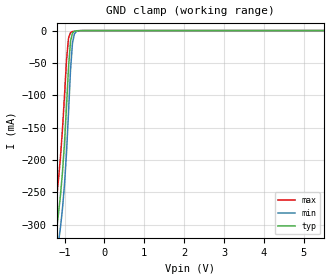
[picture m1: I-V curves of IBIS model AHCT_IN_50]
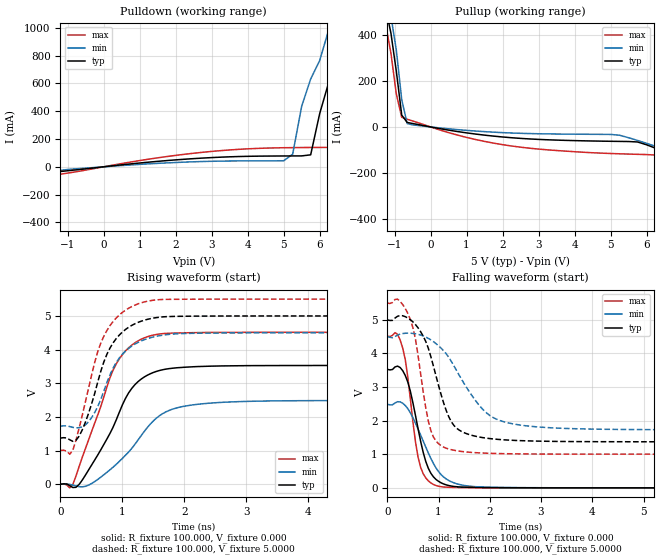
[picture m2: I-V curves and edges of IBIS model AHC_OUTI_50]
| Philips Semiconductors Inc.
| Logic Products Group
| IBIS model of 74AHCT04
| HEX INVERTER; TTL
|[Packages]:
|[Package1]: SO 14-pin (D) Package ;
|[Package2]: TSSOP 14-pin (PW) Package ;
[IBIS Ver]   3.2
[File Name]   ahct04.ibs
[File Rev]   1.4
[Date]   08-Apr-2003
[Source]   File created from simulations by LPG
   Philips Semiconductors Nijmegen
[Notes]   V1.4   Ibis model.
| Remark:
| The Power Clamp curves for the input models have been omitted since there
| is no power clamp diode.
| Revision History
| Version Date   Author/ Description
|   Editor
| 1.3   December   2000 RM   Reviewed version for IBIS 3.2
| 1.4   April   2003 RM   Updated version
[Disclaimer]
   (C) Copyright 2003 Philips Semiconductors
   All rights reserved
   Philips Semiconductors warrants and represents that the IBIS model
   identified herein is owned by Philips Semiconductors (PHILIPS). The
   model provided is not warranted as fully representing all of the
   operating characteristics and specifications of the semiconductor
   products to which the model relates.  Moreover, unless there is a
   signed, written agreement to the contrary, this IBIS model is
   furnished on an "as is" basis without support or warranty of any
   kind, either expressed or implied, regarding the use thereof, and
   PHILIPS specifically disclaims all implied warranties of
   merchantability and fitness of the model for any purpose.
   PHILIPS does not assume any liability arising out of the application
   or use of this IBIS model including infringement of patents and
   copyrights, nor does PHILIPS convey any license under its patents and
   copyrights or the rights of others.
   PHILIPS provides IBIS models as a service to our customers. You and
   your company shall not distribute, convey, sell, or give these models
   to anyone else without receiving prior written permission from
   PHILIPS.
   PHILIPS reserves the right to make changes without notice to these
   IBIS models to improve reliability, function, or design.
   Please be aware that your receipt and subsequent use of the IBIS
   information provided shall serve as acceptance of the terms and
   conditions of this agreement.  If you do not accept these terms,
   you should return or destroy the IBIS models and any other
   accompanying information immediately.
| to specify a consistent format that can be parsed by software, allowing
| simulation vendors to derive models compatible with their own products.
| One goal of this template is to represent the current state of IBIS data,
| while allowing a growth path to more complex models / methods (when deemed
| appropriate).  This would be accomplished by a revision of the base
| template, and possibly the addition of new keywords or categories.
| Another goal of this template is to ensure that it is simple enough for
| semiconductor vendors and customers to use and modify, while ensuring that
| it is rigid enough for simulation vendors to write reliable parsers.
| Finally, this template is meant to contain a complete description of the I/O
| elements on an entire component.  Consequently, several models will need to
| be defined in each file, as well as a table that equates the appropriate
| buffer to the correct pin and signal name.
| Version 3.2 of this electronic template was finalized by an industry-wide
| group of experts representing various companies and interests.  Regular
| "EIA IBIS Open Forum" meetings were held to accomplish this task.
| Commitment to Backward Compatibility.  Version 1.0 is the first valid IBIS
| ASCII file format.  It represents the minimum amount of I/O buffer
| information required to create an accurate IBIS model of common CMOS and
| bipolar I/O structures.  Future revisions of the ASCII file will add items
| considered to be "enhancements" to Version 1.0 to allow accurate modeling
| of new, or other I/O buffer structures.  Consequently, all future revisions
| will be considered supersets of Version 1.0, allowing backward
| compatibility.  In addition, as modeling platforms develop support for
| revisions of the IBIS ASCII template, all previous revisions of the template
| must also be supported.
| Version 1.1 update.  The file "ver1_1.ibs" is conceptually the same as the
| 1.0 version of the IBIS ASCII format (ver1_0.ibs).  However, various
| comments have been added for further clarification.
| Version 2.0 update.  The file "ver2_0.ibs" maintains backward compatibility
| with Versions 1.0 and 1.1.  All new keywords and elements added in Version
| 2.0 are optional.  A complete list of changes to the specification is in the
| IBIS Version 2.0 Release Notes document ("ver2_0.rn").
| Version 2.1 update.  The file "ver2_1.ibs" contains clarification text
| changes, corrections, and two additional waveform parameters beyond
| Version 2.0.
| Version 3.0 update.  The file "ver3_0.ibs" adds a number of new keywords
| and functionality.  A complete list of functions can be found on eda.org
| under /pub/ibis/birds/birddir.txt showing the approved Buffer Issue
| Resolution Documents (BIRDs) that have been approved for Version 3.0.
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[Component]   74AHCT04_1
[Manufacturer]   Philips Semiconductors Inc.
[Package]
|   typ   min   max
R_pkg   4.54E-02   4.18E-02   5.01E-02
L_pkg   2.31E-09   1.63E-09   3.26E-09
C_pkg   0.565E-12  0.437E-12  0.736E-12
[Pin] signal_name   model_name   R_pin   L_pin   C_pin
   1   1A   AHCT_IN_50 4.18E-02 3.26E-09 0.675E-12
   2   1Y#   AHC_OUTI_50 5.01E-02 2.30E-09 0.574E-12
   3   2A   AHCT_IN_50 4.52E-02 1.71E-09 0.467E-12
   4   2Y#   AHC_OUTI_50 4.38E-02 1.63E-09 0.437E-12
   5   3A   AHCT_IN_50 4.52E-02 1.71E-09 0.465E-12
   6   3Y#   AHC_OUTI_50 5.01E-02 2.30E-09 0.573E-12
   7   GND   GND 4.18E-02 3.26E-09 0.736E-12
   8   4Y#   AHC_OUTI_50 4.18E-02 3.26E-09 0.736E-12
   9   4A   AHCT_IN_50 5.01E-02 2.30E-09 0.573E-12
   10   5Y#   AHC_OUTI_50 4.52E-02 1.71E-09 0.465E-12
   11   5A   AHCT_IN_50 4.38E-02 1.63E-09 0.437E-12
   12   6Y#   AHC_OUTI_50 4.52E-02 1.71E-09 0.467E-12
   13   6A   AHCT_IN_50 5.01E-02 2.30E-09 0.574E-12
   14   VCC   POWER 4.18E-02 3.26E-09 0.736E-12
|   Info for  TSSOP 14-pin (PW) Package
[Component]   74AHCT04_2
[Manufacturer]   Philips Semiconductors Inc.
[Package]
|   typ   min   max
R_pkg   3.44E-02   2.80E-02   4.33E-02
L_pkg   1.83E-09   1.36E-09   2.32E-09
C_pkg   0.380E-12  0.302E-12  0.442E-12
[Pin] signal_name   model_name   R_pin   L_pin   C_pin
   1   1A   AHCT_IN_50 3.46E-02 2.32E-09 0.423E-12
   2   1Y#   AHC_OUTI_50 4.33E-02 2.04E-09 0.441E-12
   3   2A   AHCT_IN_50 2.80E-02 1.36E-09 0.307E-12
   4   2Y#   AHC_OUTI_50 2.88E-02 1.38E-09 0.302E-12
   5   3A   AHCT_IN_50 2.80E-02 1.36E-09 0.308E-12
   6   3Y#   AHC_OUTI_50 4.33E-02 2.04E-09 0.441E-12
   7   GND   GND 3.46E-02 2.32E-09 0.433E-12
   8   4Y#   AHC_OUTI_50 3.46E-02 2.32E-09 0.433E-12
   9   4A   AHCT_IN_50 4.33E-02 2.04E-09 0.441E-12
   10   5Y#   AHC_OUTI_50 2.80E-02 1.36E-09 0.308E-12
   11   5A   AHCT_IN_50 2.88E-02 1.38E-09 0.302E-12
   12   6Y#   AHC_OUTI_50 2.80E-02 1.36E-09 0.308E-12
   13   6A   AHCT_IN_50 4.33E-02 2.04E-09 0.442E-12
   14   VCC   POWER 3.46E-02 2.31E-09 0.433E-12
| Models and submodels in the file (2): AHCT_IN_50 (Input), AHC_OUTI_50 (Output)
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|   Model AHCT_IN_50
[Model]   AHCT_IN_50
Model_type   Input
Vinl =   0.8000V
Vinh =   2.0000V
C_comp   5.6pF   4.9pF   6.8pF
[Model Spec]
| Note: The input and output voltage ratings may be exceeded if the input and
|   output current ratings are observed (please refer to the data sheet)
|   Subparameter   typ   min   max
| Thresholds
Vinh   2.0   NA   NA
Vinl   0.8   NA   NA
| Overshoot
S_overshoot_high   7.0   7.0   7.0   | Static overshoot
S_overshoot_low   -0.5   -0.5   -0.5
D_overshoot_high   11.0   11.0   11.0   | Dynamic overshoot
D_overshoot_low   -0.95   -0.9   -1.0
D_overshoot_time   3n   3n   3n
|Ambient temperature:   25.0000   85.0000   -40.0000
[Temperature Range]   55.0000   110.0000   -5.0000
[Voltage Range]   5.0000V   4.5000V   5.5000V
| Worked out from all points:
|   GND clamp passes 1 mA (typ) near -0.75 V on its own axis
|Process Range   nominal   slow   fast
[GND Clamp]
| voltage   I(typ)   I(min)   I(max)
-5.5V     -4.525A    -4.549A    -4.495A
-1.3V     -373.3mA   -409.5mA   -330.1mA
-1.2V     -307.7mA   -348mA     -259.7mA
-1.1V     -253.8mA   -303.6mA   -194.6mA
-1.05V    -218.4mA   -274.7mA   -152mA
-950mV    -118.1mA   -189.3mA   -46.31mA
-900mV    -57.87mA   -127.6mA   -11.93mA
-850mV    -16.96mA   -61.59mA   -3.088mA
-800mV    -3.834mA   -19.15mA   -1.465mA
-750mV    -1.005mA   -4.867mA   -923uA
-600mV    -83.72uA   -113.1uA   -151.7uA
5.5V      58.3pA     1.82nA     103.7fA
|   Model AHC_OUTI_50
[Model]   AHC_OUTI_50
Model_type   Output
Polarity   Inverting
Vmeas =  2.5000V
Cref  = 50.0000pF
Rref  =  1.0000k
Vref  =  0.000V
C_comp   9.0pF   6.7pF   13.1pF
[Model Spec]
| Note: The input and output voltage ratings may be exceeded if the input and
|   output current ratings are observed (please refer to the data sheet)
|   Subparameter   typ   min   max
| Timing Thresholds
Vmeas   2.5   2.25   2.75
|Ambient temperature:   25.0000   85.0000   -40.0000
[Temperature Range]   55.0000   110.0000   -5.0000
[Voltage Range]   5.0000V   4.5000V   5.5000V
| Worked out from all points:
|   slope of the pulldown table from 0 to 0.75 V, typ, clamps not added: 35.9 ohm
|   slope of the pullup table from 0 to 0.75 V, typ, clamps not added: 37.2 ohm
|   rising waveform, R_fixture 100.000, V_fixture 0.000: 20-80 % time 593ps typ, 724ps min, 540ps max; typ from 0 V to 3.53 V
|   rising waveform, R_fixture 100.000, V_fixture 5.0000: 20-80 % time 427ps typ, 449ps min, 428ps max; typ from 1.37 V to 5 V
|   falling waveform, R_fixture 100.000, V_fixture 0.000: 20-80 % time 313ps typ, 464ps min, 232ps max; typ from 3.53 V to 0 V
|   falling waveform, R_fixture 100.000, V_fixture 5.0000: 20-80 % time 435ps typ, 728ps min, 292ps max; typ from 5 V to 1.37 V
|Process Range   nominal   slow   fast
[Pulldown]
| voltage   I(typ)   I(min)   I(max)
-5.5V     -304.7mA   -244.4mA   -420.6mA
-1.6V     -52.82mA   -44.3mA    -71.19mA
2.25V     54.55mA    33.73mA    90.24mA
5V        77.97mA    43.25mA    137.3mA
5.25V     78.26mA    90.83mA    138mA
5.5V      78.46mA    436mA      138.7mA
5.75V     86.23mA    632.3mA    139.2mA
6V        382.8mA    765.2mA    139.3mA
6.25V     606.6mA    985.4mA    139.5mA
6.75V     978.5mA    1.479A     593.9mA
7.25V     1.477A     1.981A     988mA
11V       5.298A     5.791A     4.82A
[Pullup]
| voltage   I(typ)   I(min)   I(max)
-6.5V     5.717A     5.741A     5.691A
-1.25V    521.9mA    583.1mA    449.8mA
-1.1V     409.1mA    483.8mA    321.7mA
-950mV    242.7mA    334.7mA    143.7mA
-800mV    51.78mA    119.1mA    42mA
-650mV    19.63mA    14.69mA    33.56mA
2V        -43.78mA   -24.8mA    -77.21mA
5V        -62.56mA   -32.65mA   -115.8mA
5.75V     -65.59mA   -58.92mA   -119.4mA
6.5V      -108.9mA   -97.5mA    -134mA
9.75V     -328.6mA   -269.4mA   -442.8mA
11V       -414.1mA   -336.1mA   -565.4mA
[Ramp]
| variable   typ   min   max
dV/dt_r   2.117V/593.251ps   1.493V/724.062ps   2.708V/539.812ps
dV/dt_f   2.177V/434.826ps   1.664V/728.595ps   2.698V/291.947ps
R_load = 100.000
[Rising Waveform]
R_fixture   = 100.000
V_fixture   = 0.000
V_fixture_min = 0.000
V_fixture_max = 0.000
| time   V(typ)   V(min)   V(max)
0s        402.7pV    18.45nV    554fV
200ps     -98.16mV   -25.59mV   -9.537mV
300ps     -9.255mV   -71.27mV   519mV
450ps     411.2mV    -30.31mV   1.297V
900ps     1.909V     590.1mV    3.574V
1.15ns    2.845V     1.063V     4.132V
1.45ns    3.282V     1.786V     4.409V
1.85ns    3.455V     2.254V     4.492V
2.65ns    3.516V     2.437V     4.511V
9.75ns    3.528V     2.488V     4.514V
[Rising Waveform]
R_fixture   = 100.000
V_fixture   = 5.0000
V_fixture_min = 4.5000
V_fixture_max = 5.5000
| time   V(typ)   V(min)   V(max)
0s        1.371V     1.726V     1.003V
150ps     1.321V     1.713V     892.4mV
300ps     1.424V     1.679V     1.657V
450ps     2.088V     1.85V      2.823V
600ps     3.022V     2.301V     3.927V
750ps     3.862V     3.023V     4.57V
1ns       4.522V     3.863V     5.106V
1.35ns    4.872V     4.292V     5.415V
2.25ns    4.995V     4.488V     5.498V
9.75ns    5V         4.5V       5.5V
[Falling Waveform]
R_fixture   = 100.000
V_fixture   = 0.000
V_fixture_min = 0.000
V_fixture_max = 0.000
| time   V(typ)   V(min)   V(max)
0s        3.528V     2.488V     4.514V
150ps     3.599V     2.526V     4.618V
250ps     3.582V     2.559V     4.402V
350ps     3.346V     2.452V     3.819V
600ps     1.761V     1.75V      915.3mV
750ps     787.3mV    1.214V     297.1mV
950ps     250.8mV    593.2mV    69.56mV
1.25ns    53.26mV    180mV      14.7mV
1.8ns     10.71mV    28.65mV    4.145mV
9.75ns    51.12nV    2.222uV    3.517nV
[Falling Waveform]
R_fixture   = 100.000
V_fixture   = 5.0000
V_fixture_min = 4.5000
V_fixture_max = 5.5000
| time   V(typ)   V(min)   V(max)
0s        5V         4.5V       5.5V
200ps     5.107V     4.548V     5.617V
400ps     5.056V     4.604V     5.192V
550ps     4.859V     4.585V     4.416V
650ps     4.648V     4.549V     3.398V
850ps     3.902V     4.403V     1.703V
1.2ns     2.113V     3.885V     1.155V
1.9ns     1.487V     2.28V      1.034V
2.5ns     1.411V     1.891V     1.013V
9.75ns    1.371V     1.726V     1.003V
